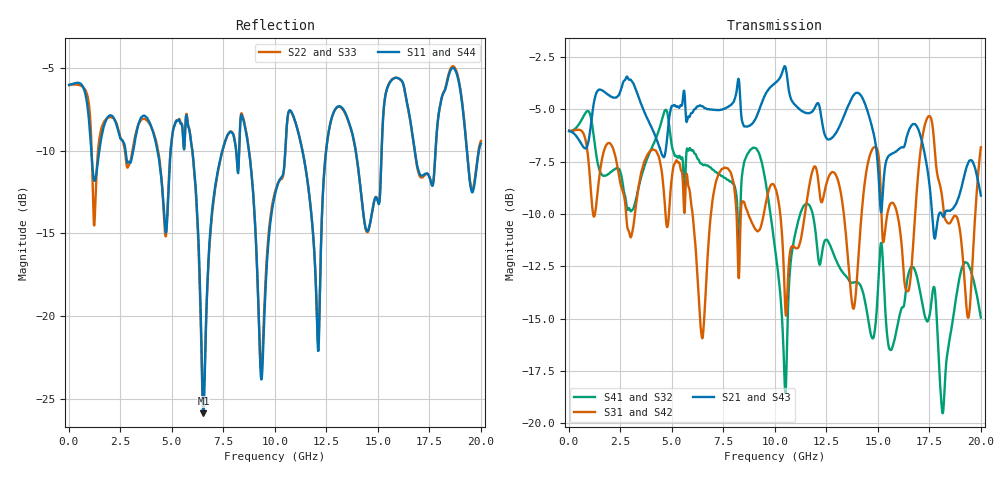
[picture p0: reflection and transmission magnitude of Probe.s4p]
! TOUCHSTONE file generated by CST MICROWAVE STUDIO
! Date and time: Thu Nov 12 08:33:28 2015
! Project name: cheetach_3_new_1inchtrace_discreteport_e3.3_waveport_new_board_vertical_coax_300mil_loss_0p01_modified_editbyxiangyang_changestackup_V2.cst
! Header version: 2015
! Port assignment regex: !\s*Touchstone port\s*([0-9]+)\s*=\s*CST MWS port\s*([0-9]+)\s*\(\"(.*)\"\)(\s*mode\s*([0-9]+))?.*
! Touchstone port assignment:
! Touchstone port 1 = CST MWS port 1 ("")
! Touchstone port 2 = CST MWS port 2 ("")
! Touchstone port 3 = CST MWS port 3 ("")
! Touchstone port 4 = CST MWS port 4 ("")
# GHz S RI R 50
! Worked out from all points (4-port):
!   1000 points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, 20 MHz to 20 GHz, reference 50 ohm
!   strongest paths, dB at 20 MHz, 5.02 GHz, 10.02 GHz, 15.02 GHz, 20 GHz:
!     S21: -6.0, -4.8, -3.7, -7.9, -9.1
!     S43: -6.0, -4.8, -3.7, -7.9, -9.1
!     S31: -6.0, -8.1, -8.7, -7.1, -6.8
!     S42: -6.0, -8.1, -8.8, -7.1, -6.8
!     S41: -6.0, -6.8, -11.7, -13.3, -14.9
!     S32: -6.0, -6.9, -11.6, -13.4, -14.9
!   lowest |S11| = -25.9 dB at 6.54 GHz (marker M1), VSWR 1.11, Z = 51.6 - j4.91 ohm
!   |S11| at or under -10 dB: 6.001 GHz to 7.459 GHz (1.458 GHz wide, 21.7 % of centre); 8.742 GHz to 10.51 GHz (1.766 GHz wide, 18.3 % of centre); 13.93 GHz to 15.18 GHz (1.258 GHz wide, 8.64 % of centre)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
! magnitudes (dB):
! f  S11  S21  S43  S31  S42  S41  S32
! 20 MHz  -6.0  -6.0  -6.0  -6.0  -6.0  -6.0  -6.0
! 5.78 GHz  -8.4  -5.4  -5.4  -8.5  -8.5  -6.9  -6.9
! 6.54 GHz  -25.9  -4.9  -4.9  -15.5  -15.2  -7.7  -7.7
! 8.42 GHz  -7.9  -5.6  -5.6  -9.4  -9.4  -8.1  -8.1
! 9.36 GHz  -23.8  -4.7  -4.7  -10.5  -10.4  -7.5  -7.5
! 10.72 GHz  -7.6  -4.3  -4.3  -12.0  -12.0  -12.9  -12.8
! 20 GHz  -9.6  -9.1  -9.1  -6.8  -6.8  -14.9  -14.9
